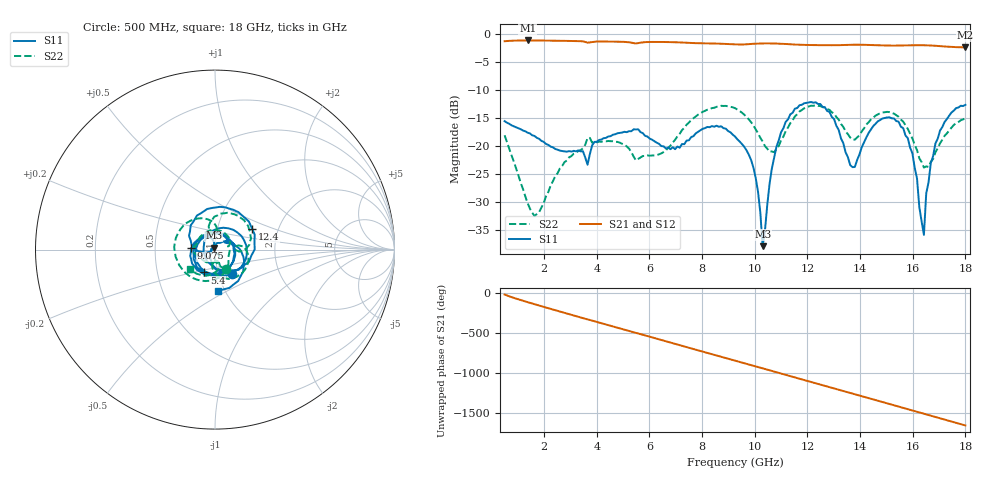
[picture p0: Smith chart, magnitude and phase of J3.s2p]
!Agilent Technologies,N5230C,MY49001096,A.09.42.15
!Agilent N5230C: A.09.42.15
!Date: Thursday, June 29, 2023 08:12:17
!Correction: S11(Full 2 Port(1,2))
!S21(Full 2 Port(1,2))
!S12(Full 2 Port(1,2))
!S22(Full 2 Port(1,2))
!S2P File: Measurements: S11, S21, S12, S22:
# Hz S  dB  R 50
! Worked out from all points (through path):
!   201 points, 500 MHz to 18 GHz, reference 50 ohm
!   highest |S21| = -1.19 dB at 1.375 GHz (marker M1); lowest = -2.4 dB at 18 GHz (marker M2)
!   group delay of S21, straight-line fit = 256 ps
!   lowest |S11| = -37.9 dB at 10.3 GHz (marker M3), VSWR 1.03, Z = 49.3 + j1.04 ohm
!   |S11| at or under -10 dB: start of sweep to end of sweep
!   |S22| runs from -32.5 to -12.8 dB; largest |S21 - S12| = 0.0013
!   S11 on the Smith chart (normalised r, x): 500 MHz: 1.16, -0.32; 5.4 GHz: 0.86, -0.22; 9.075 GHz: 0.77, +0.01; 12.4 GHz: 1.47, +0.35; 18 GHz: 0.93, -0.46
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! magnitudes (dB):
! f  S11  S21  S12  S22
! 500 MHz  -15.6  -1.3  -1.3  -18.1
! 1.375 GHz  -17.7  -1.2  -1.2  -30.2
! 1.812 GHz  -18.7  -1.2  -1.2  -31.8
! 3.475 GHz  -21.0  -1.4  -1.4  -20.4
! 3.65 GHz  -23.4  -1.6  -1.6  -18.6
! 5.4 GHz  -17.1  -1.7  -1.7  -21.9
! 6.362 GHz  -19.6  -1.5  -1.5  -21.5
! 9.075 GHz  -17.6  -1.8  -1.8  -13.0
! 9.25 GHz  -18.3  -1.9  -1.9  -13.3
! 9.95 GHz  -23.9  -1.8  -1.8  -16.4
! 10.3 GHz  -37.9  -1.7  -1.7  -19.2
! 10.65 GHz  -24.0  -1.7  -1.7  -21.0
! 11 GHz  -17.6  -1.8  -1.8  -19.0
! 12.22 GHz  -12.3  -2.0  -2.0  -12.9
! 12.4 GHz  -12.5  -2.0  -2.0  -12.9
! 13.71 GHz  -23.8  -2.0  -2.0  -18.9
! 15.11 GHz  -14.9  -2.1  -2.1  -14.0
! 15.99 GHz  -21.3  -2.0  -2.0  -18.7
! 16.43 GHz  -35.9  -2.0  -2.0  -23.9
! 16.51 GHz  -28.5  -2.1  -2.1  -23.7
! 16.86 GHz  -19.6  -2.1  -2.1  -21.2
! 18 GHz  -12.7  -2.4  -2.4  -15.1
